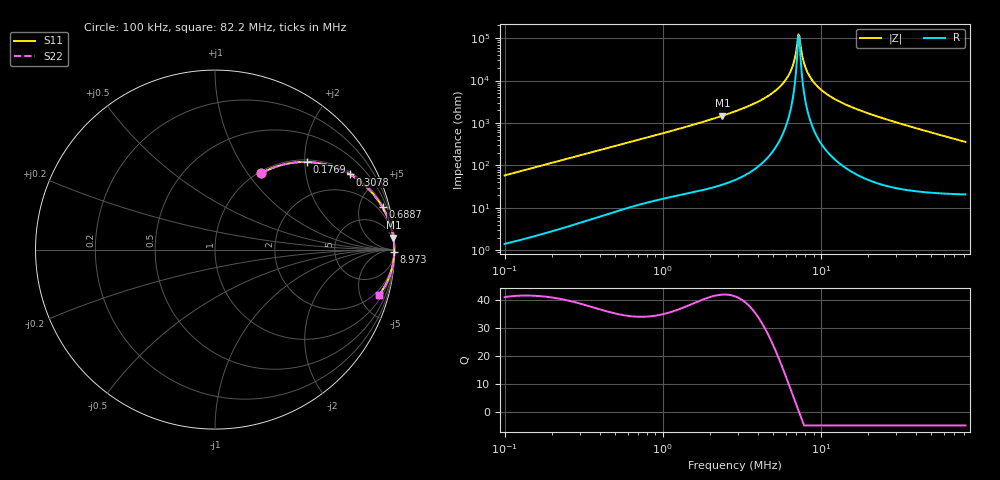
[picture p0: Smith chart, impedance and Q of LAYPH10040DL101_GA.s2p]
! LAYPH10040DL101_GA  S-PARAMETER MODEL  ( General Type )
! Model Generated by TAIYO YUDEN Corporation (http://www.ty-top.com)
! Version 1.0
! TAIYO YUDEN Control No. 180920NI43SB-FBB
! Copyright(c) 2018 TAIYO YUDEN CO.,LTD. All Rights Reserved.
! Product Description (link to TY-COMPAS)
! https://ds.yuden.co.jp/TYCOMPAS/or/detail?pn=LAYPH10040DL101MGA&u=M
! Products Name : Inductors
! Characteristics :
!  Inductance : 100 uH , SRF(min) : -Hz , DC Resistance(max) : 0.342 Ohm
!  Rated Current : Saturation :1.1 A , Temp Rise : 0.59 A (25 degC)
!  Case Size : 10.1 x 10.0 / 0.398 x 0.394 [mm/inch] , Thickness : 4 / 0.157 [mm/inch]
!  (Conditions: Temperature = 25 degC , DC Bias Current/Voltage = 0A / 0V)
! External Node Assignments :
!  1  o---GGG---o  2
! GND o---------o GND
! Frequency Range : 0.1MHz  -  82.198079MHz  [ 402 STEP ]
# MHz S RI R 50
! Freq[MHz].  S11 Real  S11 Imag  S21 Real  S21 Imag  S12 Real  S12 Imag  S22 Real  S22 Imag
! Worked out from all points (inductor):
!   401 points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, 100 kHz to 82.2 MHz, reference 50 ohm
!   read as one part in series: L = 92.6 uH near 103.4 kHz
!   highest Q = 41.9 at 2.384 MHz (marker M1), where L = 98.8 uH
!   self-resonance near 7.215 MHz
!   S11 on the Smith chart (normalised r, x): 100 kHz: 1.03, +1.17; 176.9 kHz: 1.05, +2.05; 307.8 kHz: 1.09, +3.55; 688.7 kHz: 1.23, +7.87; 8.973 MHz: open; 82.2 MHz: 1.42, -7.17
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0.1  0.2591 0.4261  0.7409 -0.4261  0.7409 -0.4261  0.2591 0.4261
0.176914  0.5124 0.4879  0.4876 -0.4879  0.4876 -0.4879  0.5124 0.4879
0.307779  0.7531 0.4184  0.2469 -0.4184  0.2469 -0.4184  0.7531 0.4184
0.688688  0.9332 0.2353  0.0668 -0.2353  0.0668 -0.2353  0.9332 0.2353
0.947281  0.9623 0.1767  0.0377 -0.1767  0.0377 -0.1767  0.9623 0.1767
2.383813  0.9939 0.067  0.00613 -0.067  0.00613 -0.067  0.9939 0.067
2.867021  0.9959 0.0529  0.0041 -0.0529  0.0041 -0.0529  0.9959 0.0529
4.361237  0.9984 0.0265  0.00157 -0.0265  0.00157 -0.0265  0.9984 0.0265
5.609408  0.9991 0.013  0.000935 -0.013  0.000935 -0.013  0.9991 0.013
6.523811  0.9992 0.00535  0.000776 -0.00535  0.000776 -0.00535  0.9992 0.00535
6.746456  0.9992 0.00367  0.000762 -0.00367  0.000762 -0.00367  0.9992 0.00367
7.094751  0.9992 0.00116  0.000753 -0.00116  0.000753 -0.00116  0.9992 0.00116
7.2148  0.9992 0.000323  0.000754 -0.000323  0.000754 -0.000323  0.9992 0.000323
7.461027  0.9992 -0.00135  0.000762 0.00135  0.000762 0.00135  0.9992 -0.00135
7.846213  0.9992 -0.00386  0.000787 0.00386  0.000787 0.00386  0.9992 -0.00386
8.113989  0.9992 -0.00554  0.000813 0.00554  0.000813 0.00554  0.9992 -0.00554
8.824095  0.9991 -0.00976  0.000911 0.00976  0.000911 0.00976  0.9991 -0.00976
8.973406  0.9991 -0.0106  0.000937 0.0106  0.000937 0.0106  0.9991 -0.0106
10.43618  0.9987 -0.0184  0.00125 0.0184  0.00125 0.0184  0.9987 -0.0184
12.98  0.998 -0.0304  0.00201 0.0304  0.00201 0.0304  0.998 -0.0304
27.15873  0.9903 -0.0851  0.00967 0.0851  0.00967 0.0851  0.9903 -0.0851
82.19808  0.9156 -0.2505  0.0844 0.2505  0.0844 0.2505  0.9156 -0.2505
